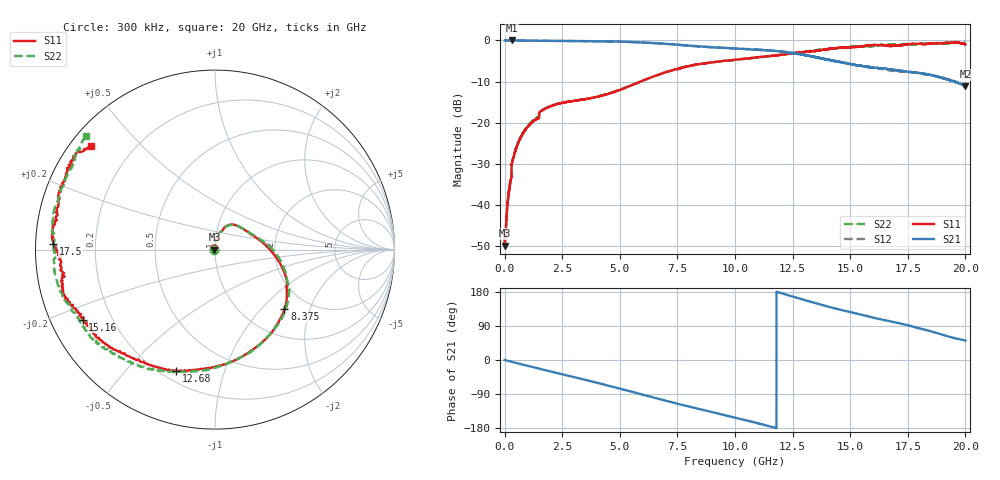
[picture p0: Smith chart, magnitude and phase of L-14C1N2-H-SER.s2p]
!{L-14C1N2}
!Johanson Technology Inc.
!www.johansontechnology.com
!Test Board Conditions:
!Substrate Type  RO4350B
!Substrate Thickness  20 mil
!Substrate Dk  3.66
!TL Type: GCPW
!TL Trace Width  36 mil
!TL Gap  12 mil
!Electrode orientation  Horizontal
!DUT TOPOLOGY	SERIES
!Mounting Pad LxW  26x36 mil
! Created Sun Jun 20 12:53:04 2021
# hz S ma R 50
! 2 Port Network Data from SP1.SP block
! freq  magS11  angS11  magS21  angS21  magS12  angS12  magS22  angS22
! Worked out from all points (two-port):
!   20001 points, 300 kHz to 20 GHz, reference 50 ohm
!   highest |S21| = -0.02 dB at 308.3 MHz (marker M1); lowest = -11.1 dB at 20 GHz (marker M2)
!   |S21| within 3 dB of the highest: start of sweep to 12.37 GHz; 12.38139 GHz to 12.39054 GHz (9.141 MHz wide, 0.0738 % of centre)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
!   lowest |S11| = -49.8 dB at 1.3 MHz (marker M3), VSWR 1.01, Z = 49.7 - j0.00731 ohm
!   |S11| at or under -10 dB: start of sweep to 5.906 GHz; 5.907782 GHz to 5.909764 GHz (1.982 MHz wide, 0.0335 % of centre)
!   |S22| runs from -50.0 to -0.4 dB; largest |S21 - S12| = 0.016
!   S11 on the Smith chart (normalised r, x): 300 kHz: 0.99, +0.00; 8.375 GHz: 1.52, -1.37; 12.68 GHz: 0.26, -0.70; 15.16 GHz: 0.10, -0.25; 17.5 GHz: 0.05, +0.02; 20 GHz: 0.06, +0.36
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300000  0.003869 170.6  0.9977 0.0  0.9947 -0.0  0.00316 -178.3
1300000  0.003218 -178.7  0.9967 -0.0  0.9968 -0.0  0.003305 177.1
1.633e8  0.01275 100.9  0.997 -2.5  0.9973 -2.5  0.01326 98.8
3.083e8  0.03097 89.9  0.9978 -4.8  0.9962 -4.8  0.03147 89.1
4.163e8  0.04103 86.9  0.9976 -6.5  0.9961 -6.4  0.0418 86.2
6.943e8  0.06572 81.4  0.9952 -10.7  0.9962 -10.7  0.06714 80.4
1.6003e9  0.1396 66.2  0.9892 -24.4  0.989 -24.4  0.1407 64.2
3.3343e9  0.1897 39.6  0.9804 -49.9  0.9799 -49.9  0.191 39.7
5.0343e9  0.2525 12.4  0.9646 -76.1  0.9635 -76.1  0.2538 13.9
6.6673e9  0.382 -14.0  0.921 -102.3  0.9177 -102.2  0.381 -11.8
8.3753e9  0.5102 -40.6  0.8489 -128.3  0.8451 -128.2  0.5109 -38.7
1.00003e10  0.5817 -64.0  0.7979 -151.8  0.7964 -151.7  0.579 -62.9
1.14703e10  0.6433 -86.1  0.7547 -174.4  0.7554 -174.2  0.6418 -84.5
1.26773e10  0.7081 -107.7  0.6871 164.3  0.6969 164.3  0.703 -105.2
1.33343e10  0.7401 -120.1  0.6389 152.9  0.6431 152.5  0.7485 -116.3
1.51563e10  0.8337 -152.1  0.5074 124.3  0.5052 123.4  0.838 -142.2
1.59853e10  0.8777 -162.7  0.4681 112.0  0.4696 111.9  0.8549 -155.3
1.66673e10  0.8519 -169.9  0.4461 103.3  0.4327 103.6  0.8935 -165.4
1.75023e10  0.9006 178.0  0.4167 91.5  0.4146 91.6  0.8917 -176.8
1.85303e10  0.9106 163.2  0.379 75.3  0.3763 75.6  0.9219 165.9
1.95323e10  0.9366 148.1  0.3153 57.7  0.3173 58.9  0.9347 145.4
2e10  0.8997 140.2  0.278 51.5  0.2721 51.8  0.9581 138.4
